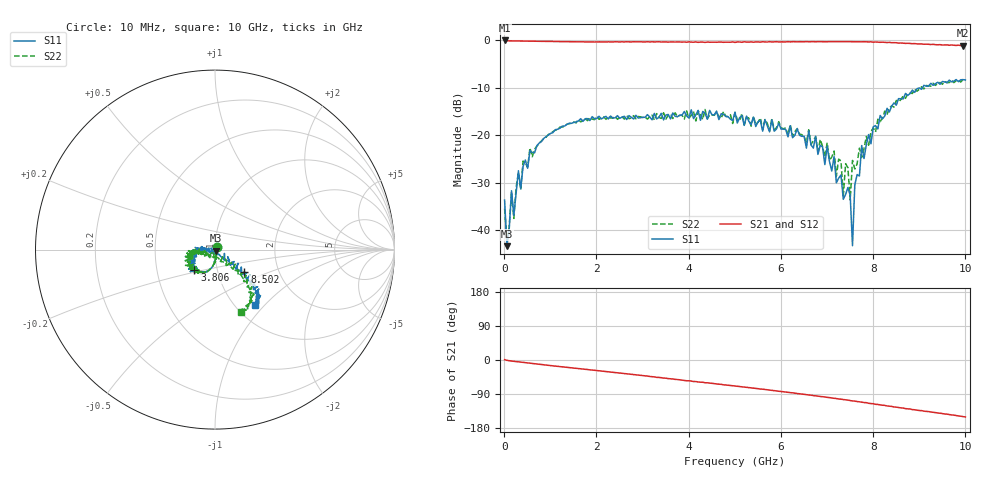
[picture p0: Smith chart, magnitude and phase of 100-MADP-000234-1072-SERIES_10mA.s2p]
!Agilent Technologies,E8364C,MY48140145,A.09.42.15
!Agilent E8364C: A.09.42.15
!Date: Wednesday, December 02, 2020 08:31:30
!Correction: S11(Full 2 Port(1,2))
!S21(Full 2 Port(1,2))
!S12(Full 2 Port(1,2))
!S22(Full 2 Port(1,2))
!S2P File: Measurements: S11, S21, S12, S22:
# Hz S  dB  R 50
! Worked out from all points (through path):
!   201 points, 10 MHz to 10 GHz, reference 50 ohm
!   highest |S21| = -0.04 dB at 10 MHz (marker M1); lowest = -1.1 dB at 9.95 GHz (marker M2)
!   group delay of S21, straight-line fit = 41 ps
!   lowest |S11| = -43.4 dB at 59.95 MHz (marker M3), VSWR 1.01, Z = 50.4 - j0.527 ohm
!   |S11| at or under -10 dB: start of sweep to 9.071 GHz
!   |S22| runs from -42.0 to -8.3 dB; largest |S21 - S12| = 0.025
!   S11 on the Smith chart (normalised r, x): 10 MHz: 1.02, +0.03; 3.806 GHz: 0.78, -0.18; 8.502 GHz: 1.34, -0.35; 10 GHz: 1.22, -0.89
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1e7  -33.67 53.1  -0.04 1.0  -0.03 -0.5  -35.46 48.4
5.995e7  -43.37 -50.3  -0.13 -0.9  -0.12 -1.1  -42.00 -58.0
1.5985e8  -31.70 -73.0  -0.14 -2.7  -0.13 -2.7  -31.93 -71.2
2.098e8  -36.88 -59.5  -0.15 -3.4  -0.14 -3.5  -37.54 -70.5
3.097e8  -27.48 -83.5  -0.17 -4.9  -0.18 -4.9  -27.81 -78.9
5.5945e8  -23.24 -91.9  -0.21 -8.6  -0.22 -8.5  -22.69 -89.1
1.7083e9  -17.09 -118.0  -0.33 -24.1  -0.32 -23.8  -16.90 -116.7
3.35665e9  -16.22 -136.7  -0.32 -46.0  -0.34 -46.2  -16.28 -126.4
3.8062e9  -15.77 -134.7  -0.37 -52.3  -0.34 -52.2  -15.83 -135.3
5.005e9  -15.16 -150.0  -0.46 -68.7  -0.40 -68.6  -15.21 -167.4
6.7033e9  -22.70 175.0  -0.29 -94.0  -0.27 -93.6  -21.12 177.9
7.3027e9  -28.39 -168.2  -0.30 -103.4  -0.30 -103.7  -25.43 -122.4
7.35265e9  -33.50 -99.2  -0.31 -104.4  -0.26 -104.0  -32.80 -134.2
7.45255e9  -31.02 -107.1  -0.30 -105.7  -0.29 -106.1  -26.82 -87.8
7.5025e9  -32.69 -54.8  -0.31 -107.2  -0.27 -106.6  -33.60 -109.8
7.55245e9  -43.28 -109.2  -0.31 -107.8  -0.31 -108.0  -25.31 -96.1
7.6024e9  -30.46 -54.2  -0.31 -108.6  -0.30 -108.6  -27.12 -76.2
7.75225e9  -22.18 -47.2  -0.33 -111.3  -0.30 -111.0  -24.69 -42.9
8.35165e9  -15.11 -33.5  -0.46 -121.9  -0.48 -121.9  -14.23 -48.0
8.5015e9  -13.68 -37.6  -0.52 -124.4  -0.56 -124.7  -12.68 -45.9
9.95005e9  -8.29 -51.3  -1.13 -149.5  -1.15 -149.3  -8.26 -67.9
1e10  -8.35 -54.1  -1.11 -150.3  -1.11 -150.4  -8.46 -67.6
